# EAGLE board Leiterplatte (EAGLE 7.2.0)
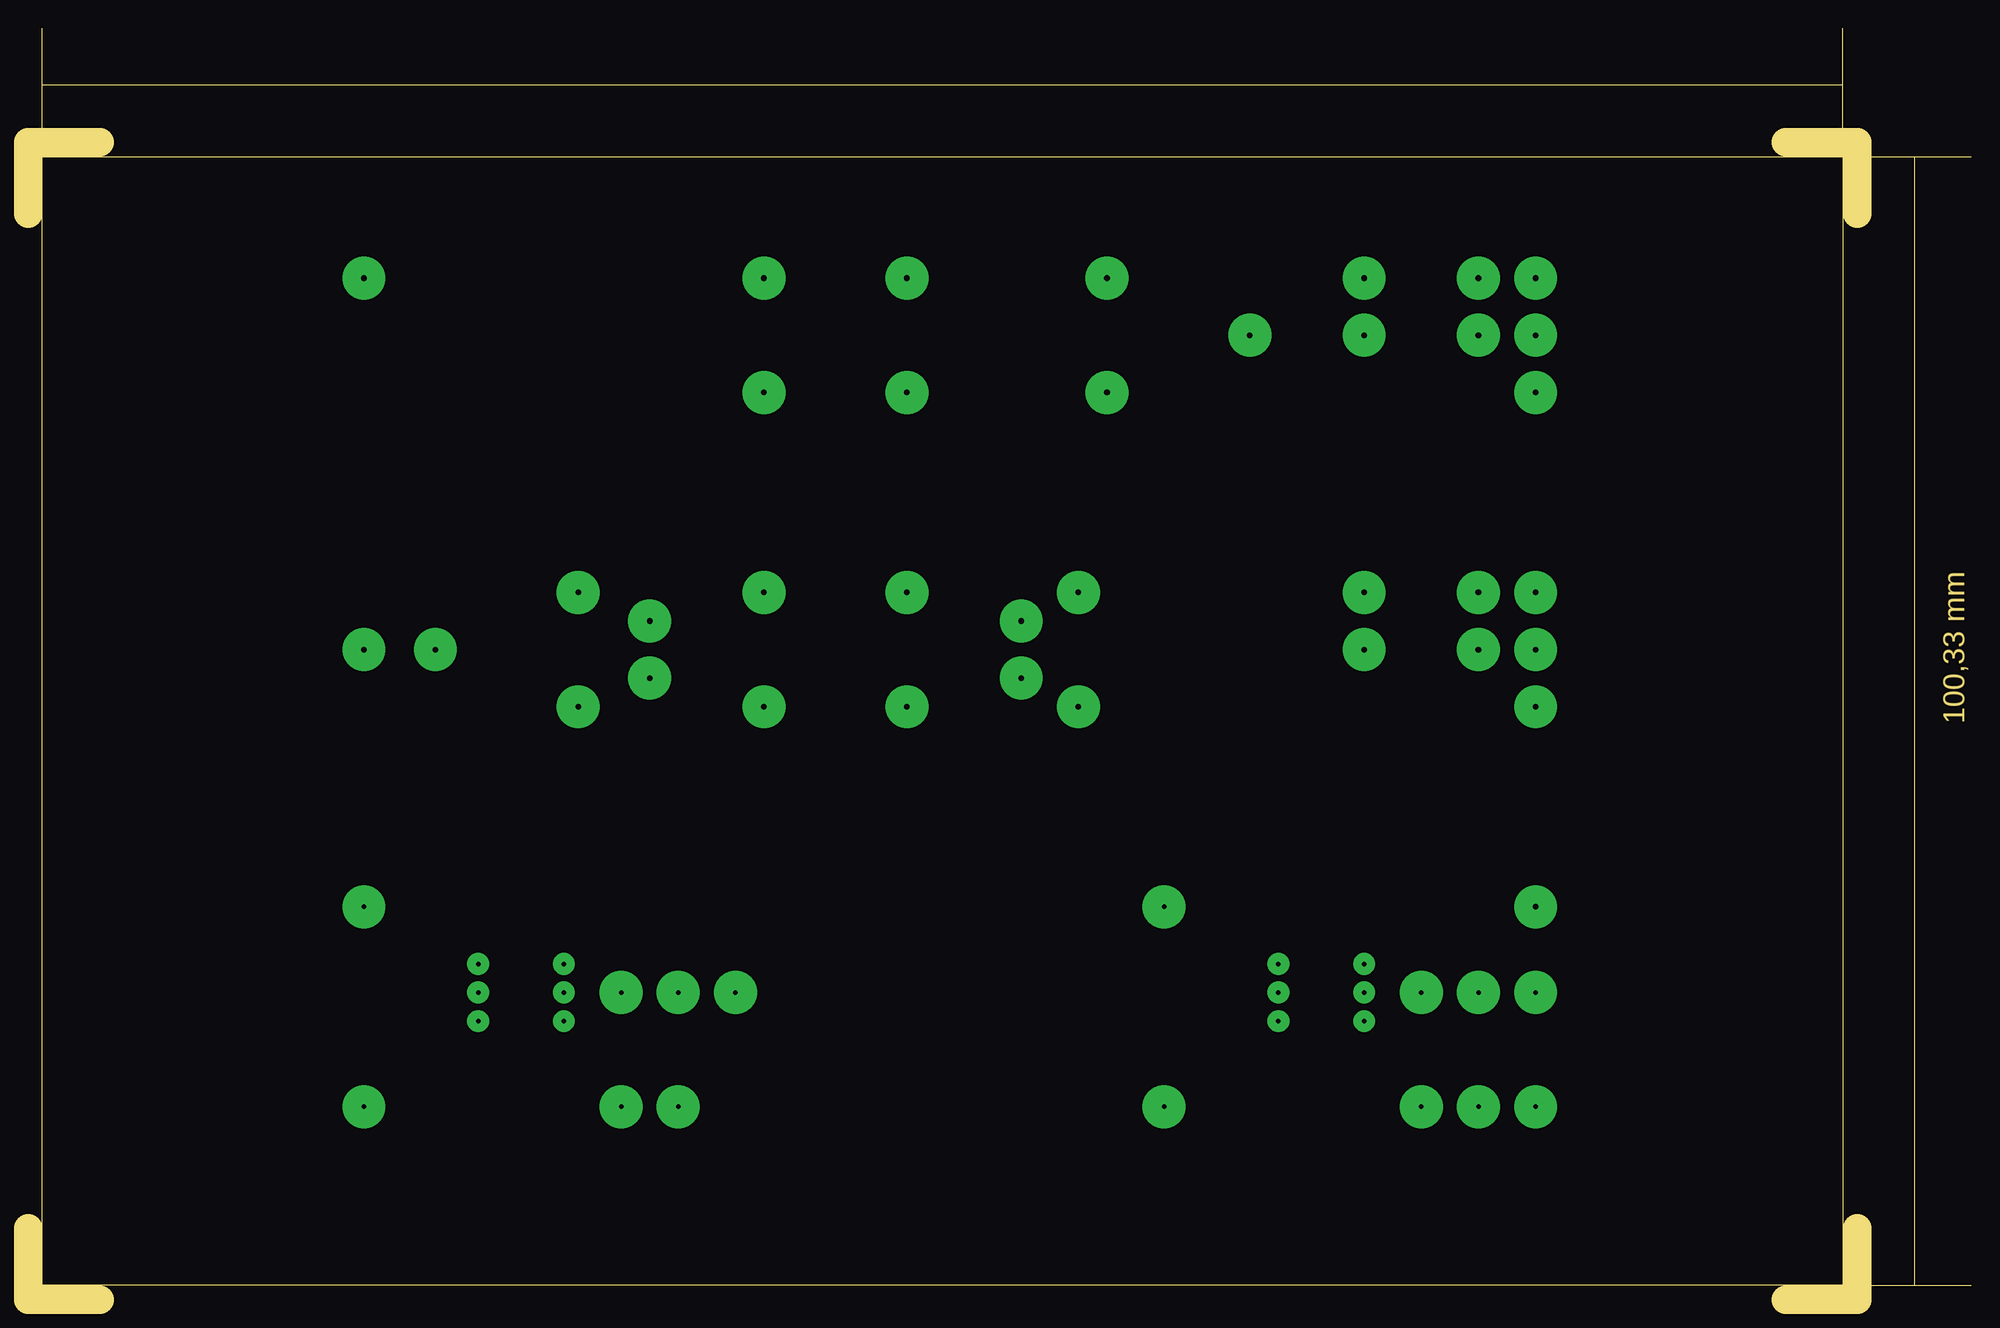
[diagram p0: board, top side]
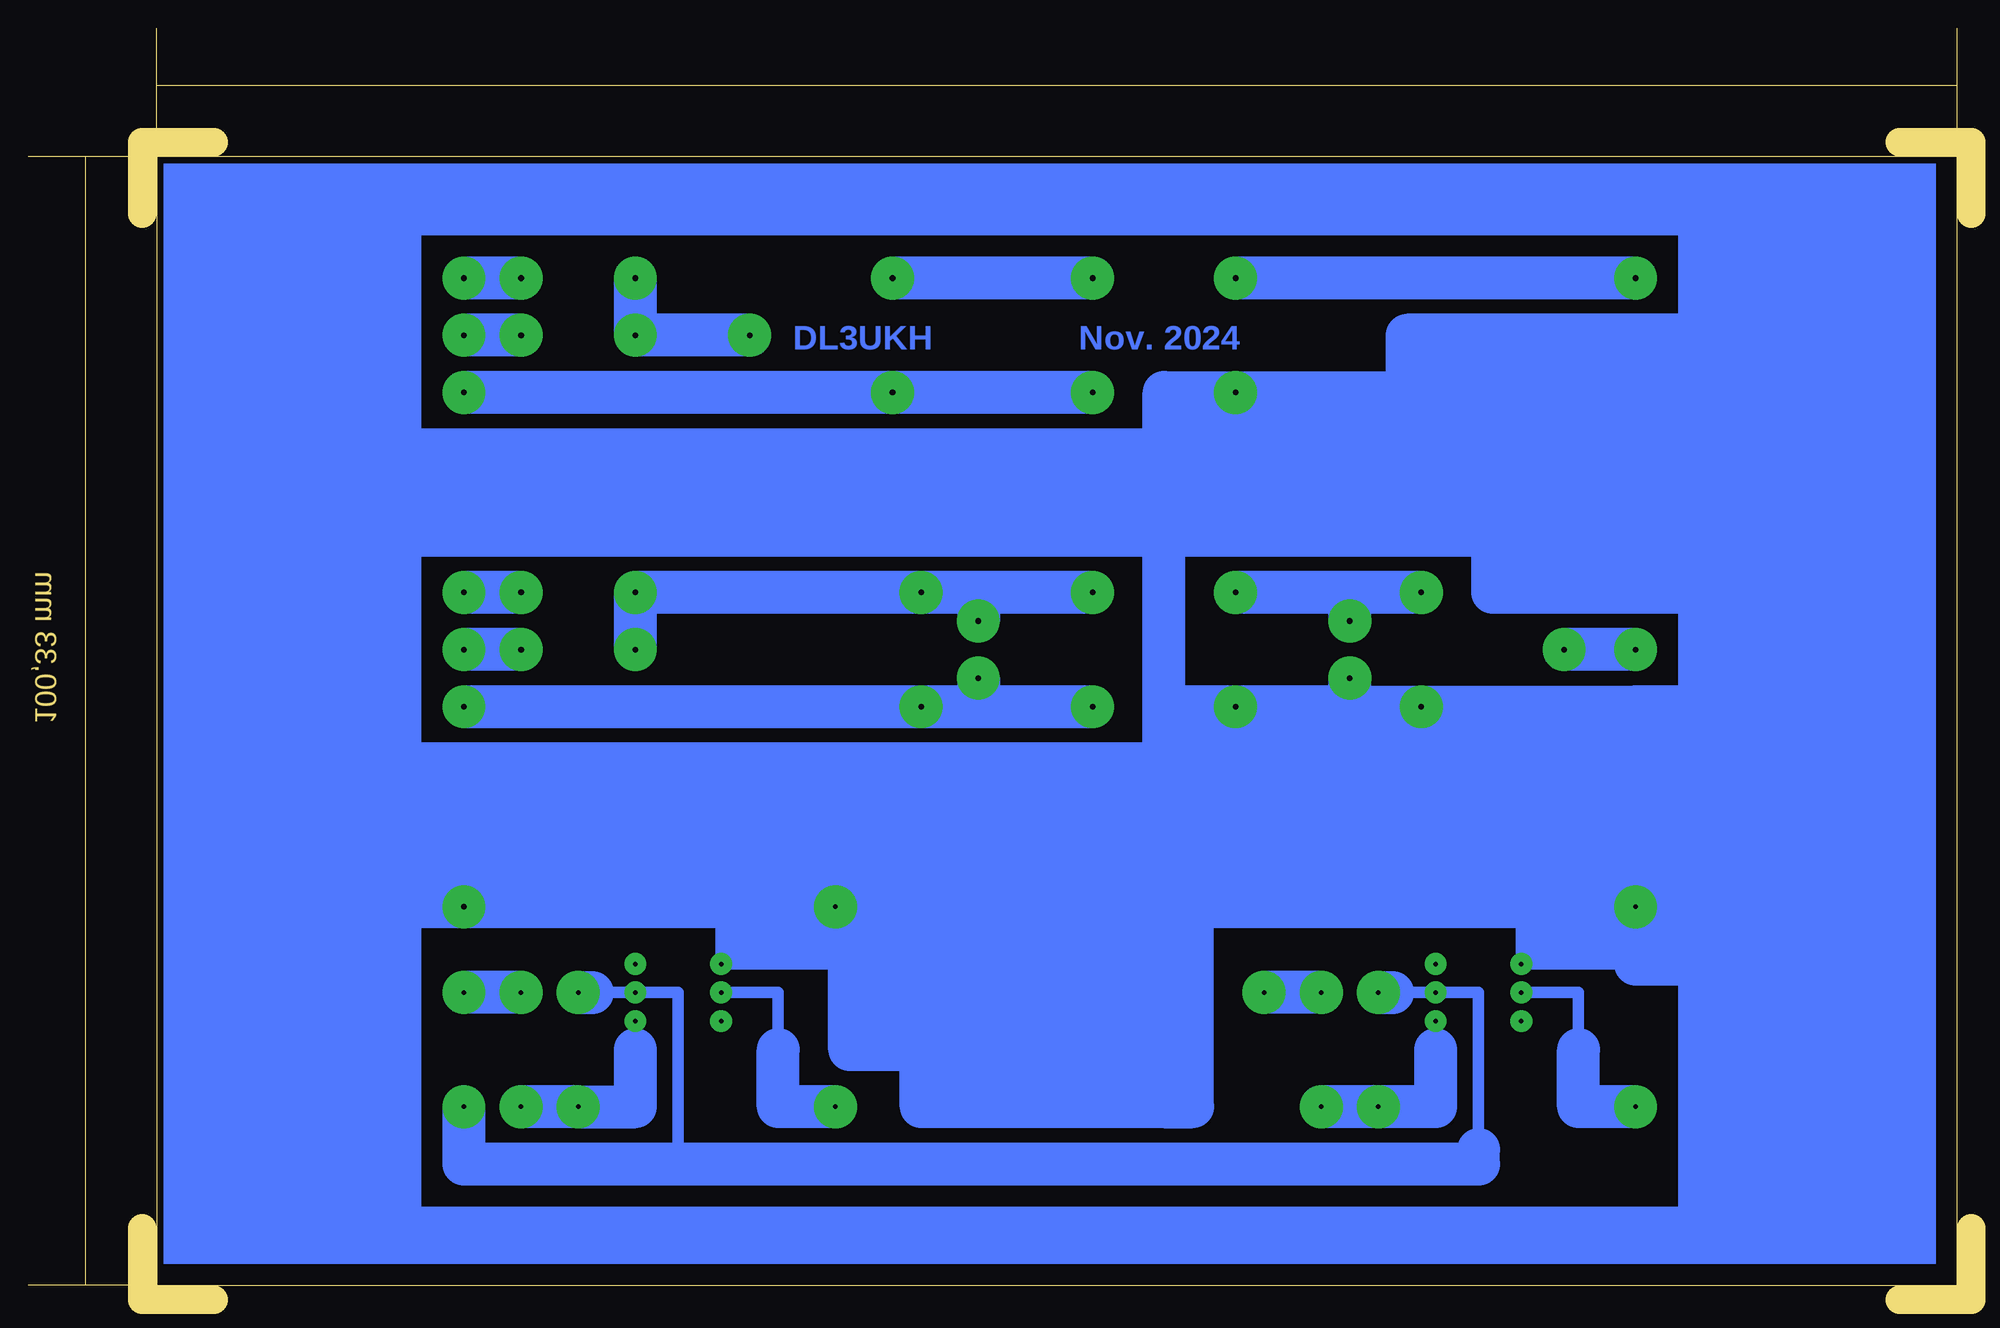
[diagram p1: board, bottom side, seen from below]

Size 172.72 x 113.03 mm. Coordinates in mm from the lower left corner, seen from the top.
Outline: 1.27,101.6 1.27,1.27 161.29,1.27
Outline: 1.27,101.6 161.29,101.6
Outline: 161.29,101.6 161.29,1.27
Outline: 0,6.35 0,0 6.35,0
Outline: 0,97.79 0,99.06
Outline: 0,99.06 0,102.87 6.35,102.87
Outline: 0,99.06 0,96.52
Outline: 156.21,102.87 162.56,102.87 162.56,96.52
Outline: 162.56,6.35 162.56,0 156.21,0
Outline: 1.27,101.6 1.27,107.95
Outline: 1.27,107.95 1.27,113.03
Outline: 161.29,101.6 161.29,107.95
Outline: 161.29,107.95 161.29,113.03
Outline: 161.29,107.95 1.27,107.95
Outline: 161.29,101.6 167.64,101.6
Outline: 167.64,101.6 172.72,101.6
Outline: 161.29,1.27 167.64,1.27
Outline: 167.64,1.27 172.72,1.27
Outline: 167.64,101.6 167.64,1.27
Copper layers 16: Bottom 0.035mm
Design rules "default": minimum track width 10mil, minimum drill 24mil, track to track 8mil, track to pad 8mil, pad to pad 8mil, via to via 8mil, smd to smd 8mil, copper to edge 40mil, drill to drill 8mil, minimum pad ring 10mil, minimum via ring 8mil, stop-mask expansion 4mil, vias tented up to drill 0mil, thermal gap 10mil

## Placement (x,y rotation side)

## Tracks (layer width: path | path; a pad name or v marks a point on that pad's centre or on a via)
S$1  (via drill 0.4 pad 1.93, 0.4 pad 3.81)
  Bottom 1.016: v40.01,27.3 34.93,27.3 34.93,22.22
  Bottom 3.81: v29.84,17.14 34.93,17.14 34.93,22.22
S$2  (via drill 0.4 pad 3.81)
  other vias: 128.91,27.3
S$3  (via drill 0.5 pad 3.81)
  Bottom 3.81: v78.1,90.8 88.27,90.8 v95.88,90.8
S$4  (via drill 0.4 pad 1.93)
  other vias: 40.01,24.77
S$5  (via drill 0.4 pad 1.93)
  other vias: 47.62,29.84
S$6  (via drill 0.4 pad 1.93, 0.4 pad 3.81)
  Bottom 1.016: 122.55,27.3 v118.74,27.3 114.94,27.3 114.94,12.06 | 51.44,27.3 v47.62,27.3 43.82,27.3 43.82,13.33 | 43.82,12.06 114.94,12.06 | 114.94,12.06 133.99,12.06
  Bottom 3.81: v133.99,17.14 133.99,12.06 43.82,12.06 43.82,13.33 | v52.71,27.3 51.44,27.3 | v123.83,27.3 122.55,27.3
S$7  (via drill 0.5 pad 3.81)
  Bottom 3.81: v48.9,62.87 55.25,62.87 | 55.25,62.87 v65.41,62.87 | v55.25,60.33 55.25,62.87
S$8  (via drill 0.4 pad 1.93, 0.4 pad 3.81)
  Bottom 1.016: v111.12,27.3 106.05,27.3 106.05,22.22
  Bottom 3.81: v100.96,17.14 106.05,17.14 106.05,22.22
S$9  (via drill 0.4 pad 1.93)
  other vias: 111.12,24.77
S$10  (via drill 0.4 pad 1.93)
  other vias: 118.74,29.84
S$11  (via drill 0.5 pad 3.81)
  Bottom 3.81: v78.1,80.64 88.27,80.64 v95.88,80.64 v133.99,80.64
S$12  (via drill 0.4 pad 1.93, 0.4 pad 3.81)
  Bottom 1.016: v118.74,24.77 118.74,22.22
  Bottom 3.81: v128.91,17.14 v123.83,17.14 118.74,17.14 118.74,22.22
S$13  (via drill 0.4 pad 1.93, 0.4 pad 3.81)
  Bottom 1.016: v47.62,24.77 47.62,22.22
  Bottom 3.81: v57.79,17.14 v52.71,17.14 47.62,17.14 47.62,22.22
S$14  (via drill 0.4 pad 3.81)
  Bottom 3.81: v57.79,27.3 v62.87,27.3 | 128.91,27.3 v133.99,27.3
S$15  (via drill 0.5 pad 3.81)
  Bottom 3.81: v108.58,85.72 v118.74,85.72 v118.74,90.8
S$16  (via drill 0.5 pad 3.81)
  Bottom 3.81: v29.84,90.8 55.25,90.8 v65.41,90.8
S$17  (via drill 0.4 pad 1.93, 0.4 pad 3.81, 0.5 pad 3.81)
  Bottom 1.016: 29.84,31.11 29.84,29.84 v40.01,29.84 40.01,34.93 | 106.05,29.84 v111.12,29.84 | 106.05,29.84 v100.96,34.93 100.96,29.84 | 106.05,34.93 106.05,29.84 | 100.96,29.84 v111.12,29.84 | v111.12,29.84 111.12,34.93 | 100.96,29.84 93.34,29.84
  Bottom 3.81: 42.55,67.94 141.61,67.94 141.61,75.56 71.75,75.56 | v133.99,34.93 111.12,34.93 106.05,34.93 v100.96,34.93 71.75,34.93 | 55.25,52.71 v48.9,52.71 | 55.25,52.71 v65.41,52.71 | 55.25,52.71 v55.25,55.25 | 71.75,34.93 71.75,52.71 | 71.75,52.71 71.75,75.56 | 71.75,75.56 71.75,80.64 v65.41,80.64 22.22,80.64 | 55.25,34.93 69.21,34.93 | 69.21,34.93 71.75,34.93 | 55.25,34.93 55.25,52.71 | v29.84,34.93 40.01,34.93 55.25,34.93 | 71.75,34.93 71.75,22.22 | 71.75,17.14 93.34,17.14 93.34,22.22 | 93.34,22.22 93.34,29.84 93.34,33.66 | v29.84,34.93 29.84,47.62 | 29.84,47.62 133.99,47.62 | 133.99,47.62 v133.99,34.93 | v29.84,34.93 29.84,31.11 | v48.9,52.71 48.9,46.36 | v65.41,52.71 65.41,46.36 | v65.41,52.71 71.75,52.71 | 93.34,22.22 99.69,22.22 99.69,31.11 | 93.34,22.22 71.75,22.22 | 71.75,22.22 71.75,17.14 | 71.75,17.14 69.21,17.14 69.21,34.93 | v48.9,52.71 29.84,52.71 | 29.84,52.71 29.84,47.62 | 133.99,47.62 141.61,47.62 | v133.99,34.93 141.61,34.93 | 29.84,29.84 20.95,29.84 20.95,52.71 29.84,52.71 | 42.55,67.94 42.55,62.87 23.5,62.87 23.5,67.94 42.55,67.94
S$18  (via drill 0.5 pad 3.81)
  Bottom 3.81: v128.91,85.72 v133.99,85.72
S$19  (via drill 0.5 pad 3.81)
  Bottom 3.81: v128.91,90.8 v133.99,90.8
S$20
  Bottom 3.81: 24.77,85.72 50.17,85.72 50.17,78.1
S$21  (via drill 0.5 pad 3.81)
  Bottom 3.81: v128.91,57.79 v133.99,57.79
S$22  (via drill 0.5 pad 3.81)
  Bottom 3.81: v128.91,62.87 v133.99,62.87
S$23  (via drill 0.5 pad 3.81)
  Bottom 3.81: v118.74,57.79 v118.74,62.87 v93.34,62.87 88.27,62.87 | v78.1,62.87 88.27,62.87 | 88.27,62.87 v88.27,60.33
S$24
  Bottom 3.81: 49.53,83.19 48.9,83.19
S$27  (via drill 0.5 pad 3.81)
  Bottom 3.81: v78.1,52.71 88.27,52.71 | 88.27,52.71 v93.34,52.71 v133.99,52.71 | v88.27,55.25 88.27,52.71
S$30  (via drill 0.5 pad 3.81)
  Bottom 3.81: v29.84,57.79 v36.2,57.79
(copper drawn outside any net)
  shapes: Bottom area x18

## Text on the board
Bottom: Nov. 2024 | DL3UKH
Dimension: 100,33 mm
tOrigins: 160,02mm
